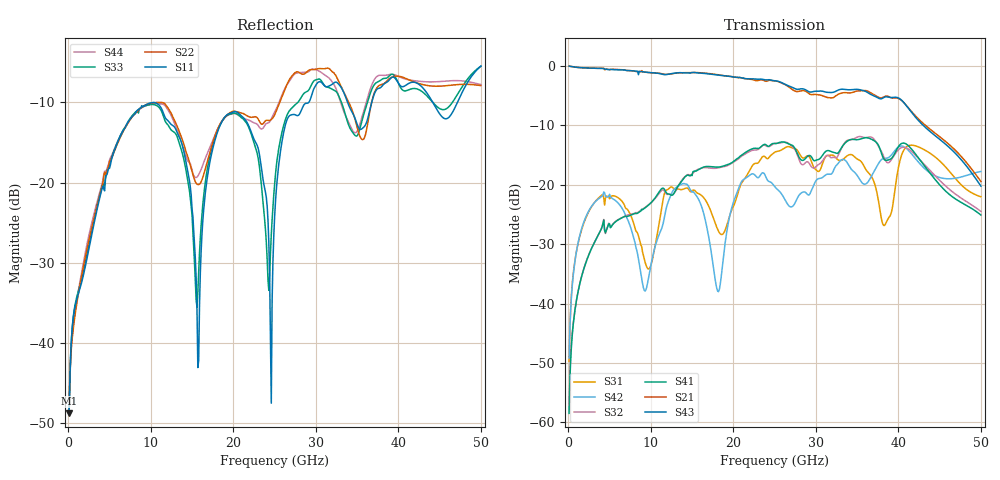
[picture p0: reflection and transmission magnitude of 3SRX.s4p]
! DAC39RF10ACK
! 256-pin FCBGA package
! Texas Instruments 8/20/2022
! Single-ended  S-parameters
! PORT#  PORT_NAME  NET_NAME
! PORT1:  xSRXN.DIEBUMP  xSRXN
! PORT2:  xSRXN.BGA  xSRXN
! PORT3:  xSRXP.DIEBUMP  xSRXP
! PORT4:  xSRXP.BGA  xSRXP
! Touchstone Ver. 1.0
! Number of ports is 4
# Hz	S	MA	R	50.000000
! SCATTERING PARAMETERS  :
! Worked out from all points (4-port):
!   500 points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, 100 MHz to 50 GHz, reference 50 ohm
!   strongest paths, dB at 100 MHz, 12.6 GHz, 25.1 GHz, 37.6 GHz, 50 GHz:
!     S43: 0.0, -1.3, -2.5, -5.4, -20.2
!     S21: 0.0, -1.3, -2.5, -5.3, -19.5
!     S41: -58.5, -21.8, -13.1, -13.4, -25.1
!     S32: -56.9, -21.7, -13.0, -13.5, -24.5
!     S42: -49.2, -21.2, -20.5, -16.4, -17.8
!     S31: -49.7, -20.4, -14.5, -22.8, -22.0
!   lowest |S11| = -48.7 dB at 100 MHz (marker M1), VSWR 1.01, Z = 50.3 + j0.186 ohm
!   |S11| at or under -10 dB: start of sweep to 10.29 GHz; 10.32 GHz to 29.13 GHz (18.8 GHz wide, 95.3 % of centre); 44.18 GHz to 47.16 GHz (2.98 GHz wide, 6.52 % of centre)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
1e8  0.003659 30.4  0.9887 -2.3  0.003155 84.7  0.001379 -99.9
     0.9965 -2.1  0.00429 24.6  0.001172 -98.1  0.003201 84.4
     0.00326 84.5  0.001421 -103.7  0.003671 30.4  0.9958 -2.3
     0.00119 -98.2  0.003483 74.6  0.9965 -2.2  0.003668 26.0
8.9e9  0.3019 -69.6  0.8937 -170.7  0.02907 -121.2  0.061 90.7
       0.9142 -170.0  0.2958 -94.6  0.06103 89.2  0.01604 -123.0
       0.03006 -122.6  0.06156 89.5  0.295 -71.3  0.8913 -172.2
       0.06224 92.1  0.0161 -125.0  0.8958 -172.3  0.2929 -96.5
1.57e10  0.007051 117.7  0.8784 62.1  0.08525 -43.5  0.1338 -32.5
         0.8798 62.3  0.09735 -130.0  0.1336 -34.7  0.07645 -8.3
         0.08464 -43.2  0.1346 -34.8  0.02078 33.5  0.8766 59.5
         0.133 -32.0  0.07733 -7.4  0.874 59.3  0.1101 -123.4
1.84e10  0.2282 -70.8  0.8356 8.7  0.03827 -159.2  0.1409 -88.4
         0.8382 8.7  0.2323 -102.4  0.139 -90.3  0.01447 64.4
         0.03871 -158.6  0.1398 -90.3  0.2296 -71.2  0.8381 6.1
         0.1415 -88.2  0.01426 57.3  0.8344 6.2  0.2323 -106.5
2.46e10  0.00423 -0.0  0.7537 -111.2  0.178 -47.0  0.2185 143.7
         0.7554 -110.9  0.2475 -113.0  0.2165 141.2  0.1048 -28.9
         0.1781 -46.9  0.2147 141.1  0.04733 14.6  0.7628 -115.0
         0.219 143.8  0.1044 -29.5  0.7606 -115.4  0.2496 -108.6
2.68e10  0.2613 -61.5  0.6611 -158.0  0.2094 -132.7  0.2191 87.1
         0.6598 -157.8  0.4399 -112.0  0.219 81.2  0.06678 -117.6
         0.2088 -133.2  0.2198 80.7  0.2809 -54.1  0.6745 -160.3
         0.2198 86.7  0.06585 -118.0  0.6761 -160.2  0.4296 -113.1
5e10  0.5323 -100.9  0.1099 137.4  0.0723 170.3  0.05916 11.6
      0.1065 136.1  0.403 -167.0  0.05559 7.0  0.133 25.1
      0.07917 173.3  0.05972 8.5  0.532 -105.9  0.09871 120.8
      0.05562 11.6  0.1294 28.6  0.0975 124.5  0.409 -169.9
